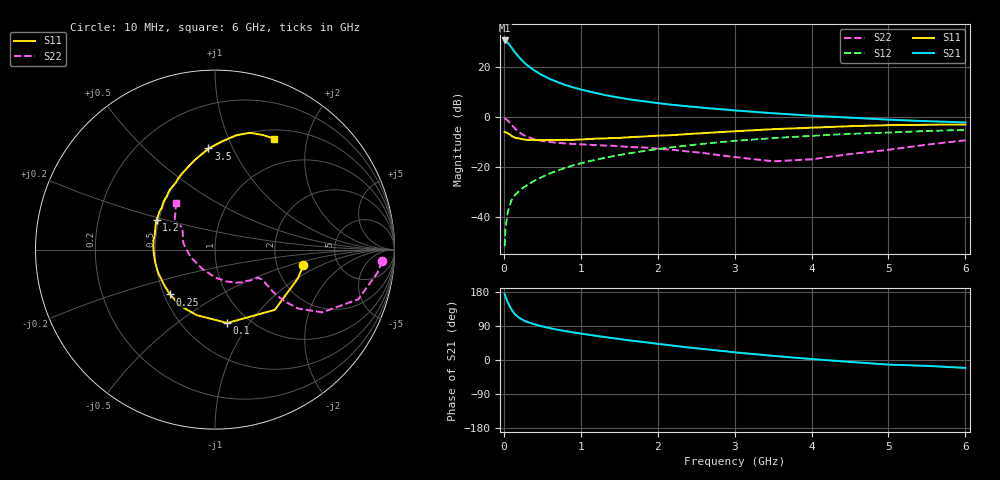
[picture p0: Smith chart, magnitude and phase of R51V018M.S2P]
! SIEMENS Small Signal Semiconductors
! BFR183
! Si NPN RF Bipolar Junction Transistor in SOT23
! VCE = 1 V  IC = 18 mA
! Common Emitter S-Parameters:  May  1996
# GHz  S  MA  R  50
!  f  S11  S21  S12  S22
! GHz  MAG  ANG  MAG  ANG  MAG  ANG  MAG  ANG
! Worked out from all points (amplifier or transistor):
!   36 points, 10 MHz to 6 GHz, reference 50 ohm
!   highest |S21| = 30.5 dB at 10 MHz (marker M1)
!   |S21| within 3 dB of that: start of sweep to 103.9 MHz
!   unconditionally stable (mu >= 1): 450.4 MHz to 2.712 GHz
!   at 250 MHz: K = 0.83, MSG = 25.2 dB, |S12| = -28.4 dB
!   at 1.4 GHz: K = 1.08, MAG = 10.3 dB, |S12| = -15.9 dB
!   at 6 GHz: K = 0.95, MSG = 1.5 dB, |S12| = -5.3 dB
!   S11 on the Smith chart (normalised r, x): 10 MHz: 2.82, -0.66; 100 MHz: 0.80, -0.79; 250 MHz: 0.54, -0.31; 1.2 GHz: 0.49, +0.19; 3.5 GHz: 0.49, +0.81; 6 GHz: 0.61, +1.48
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0.01  0.4995 -10.1  33.41 174.1  0.0026 86.4  0.9329 -4.0
0.02  0.4889 -19.2  33.09 168.0  0.0055 82.2  0.9146 -8.1
0.05  0.473 -45.2  30.43 152.3  0.0124 73.5  0.8449 -19.1
0.1  0.4145 -80.5  24.1 132.8  0.0217 66.6  0.6927 -30.3
0.15  0.3792 -105.8  18.92 119.5  0.0278 63.5  0.5688 -35.3
0.2  0.3677 -122.0  15.35 111.3  0.0327 63.2  0.4902 -36.5
0.25  0.3537 -135.1  12.69 105.2  0.0382 63.7  0.4359 -36.6
0.3  0.3455 -145.0  10.83 100.6  0.0428 64.8  0.3996 -36.0
0.4  0.3419 -158.7  8.358 94.1  0.0531 66.5  0.354 -34.4
0.5  0.3409 -168.5  6.747 88.6  0.0631 68.0  0.3283 -33.1
0.6  0.3413 -176.2  5.679 84.0  0.074 68.2  0.3133 -32.6
0.7  0.3443 177.0  4.912 79.8  0.0847 68.7  0.3018 -32.6
0.8  0.3462 171.3  4.317 76.3  0.0957 68.1  0.293 -32.9
0.9  0.3457 166.4  3.869 72.9  0.1069 67.6  0.2857 -33.2
1.1  0.3579 157.4  3.22 66.8  0.1284 66.4  0.2765 -35.8
1.2  0.3653 152.9  2.971 63.7  0.1392 65.6  0.2706 -36.9
1.6  0.3879 138.4  2.265 52.6  0.1827 61.5  0.2512 -43.7
2.2  0.4297 121.1  1.725 37.9  0.2473 54.5  0.2186 -57.7
3.5  0.5646 93.7  1.174 10.9  0.3741 36.5  0.1288 -122.7
4.5  0.6475 79.6  0.96 -5.0  0.4561 23.0  0.1798 168.9
5.5  0.6917 67.4  0.815 -15.5  0.5194 11.0  0.2775 144.0
6  0.7002 62.1  0.77 -20.9  0.5463 3.5  0.3384 129.8
